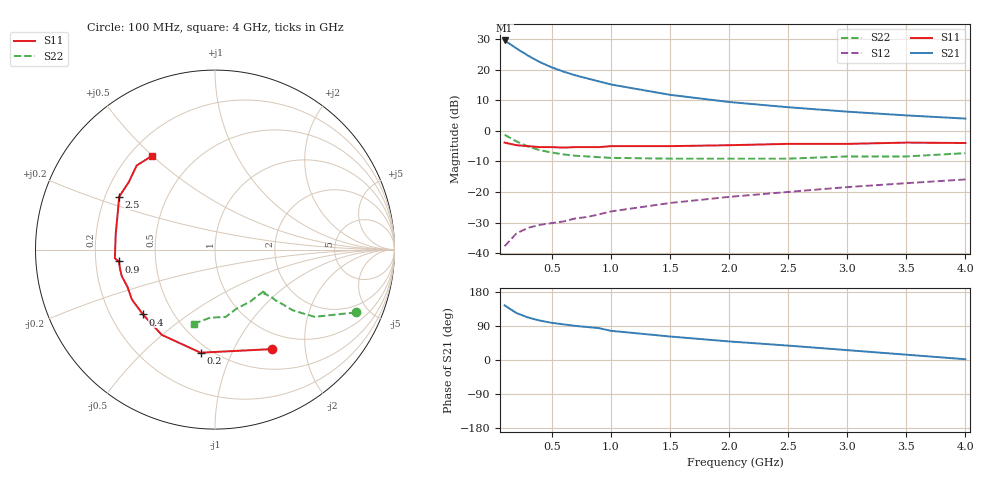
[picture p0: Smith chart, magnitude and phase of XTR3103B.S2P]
! HXTR-3103  (2N6838) Common Emitter
! Vce=10V Ic=15mA
# ghz s ma r 50
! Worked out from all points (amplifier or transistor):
!   16 points, 100 MHz to 4 GHz, reference 50 ohm
!   highest |S21| = 29.5 dB at 100 MHz (marker M1)
!   |S21| within 3 dB of that: start of sweep to 216.7 MHz
!   unconditionally stable (mu >= 1): 762.9 MHz to 2.905 GHz
!   at 300 MHz: K = 0.55, MSG = 28.1 dB, |S12| = -31.7 dB
!   at 900 MHz: K = 1.05, MAG = 20.3 dB, |S12| = -27.3 dB
!   at 4 GHz: K = 0.85, MSG = 9.9 dB, |S12| = -15.9 dB
!   S11 on the Smith chart (normalised r, x): 100 MHz: 0.77, -1.44; 200 MHz: 0.44, -0.77; 400 MHz: 0.34, -0.35; 900 MHz: 0.30, -0.06; 2.5 GHz: 0.26, +0.24; 4 GHz: 0.29, +0.50
0.1  0.64 -60.0  29.85 144.0  0.013 57.0  0.86 -24.0
0.2  0.58 -98.0  22.13 124.0  0.021 47.0  0.67 -34.0
0.3  0.56 -122.0  16.78 112.0  0.026 44.0  0.55 -38.0
0.4  0.54 -138.0  13.18 104.0  0.029 43.0  0.48 -39.0
0.5  0.54 -149.0  10.83 98.0  0.031 44.0  0.44 -40.0
0.6  0.53 -157.0  9.22 94.0  0.033 47.0  0.41 -40.0
0.7  0.54 -164.0  8.03 90.0  0.037 49.0  0.39 -41.0
0.8  0.54 -168.0  7.16 87.0  0.039 50.0  0.38 -41.0
0.9  0.54 -173.0  6.38 84.0  0.043 52.0  0.37 -42.0
1  0.56 -175.0  5.7 77.0  0.048 49.0  0.36 -39.0
1.5  0.56 171.0  3.86 62.0  0.066 54.0  0.35 -47.0
2  0.58 159.0  2.95 49.0  0.083 52.0  0.35 -56.0
2.5  0.61 151.0  2.42 38.0  0.1 51.0  0.35 -70.0
3  0.61 142.0  2.05 26.0  0.12 47.0  0.38 -81.0
3.5  0.64 133.0  1.78 14.0  0.139 44.0  0.38 -94.0
4  0.63 124.0  1.58 2.0  0.16 39.0  0.43 -106.0
